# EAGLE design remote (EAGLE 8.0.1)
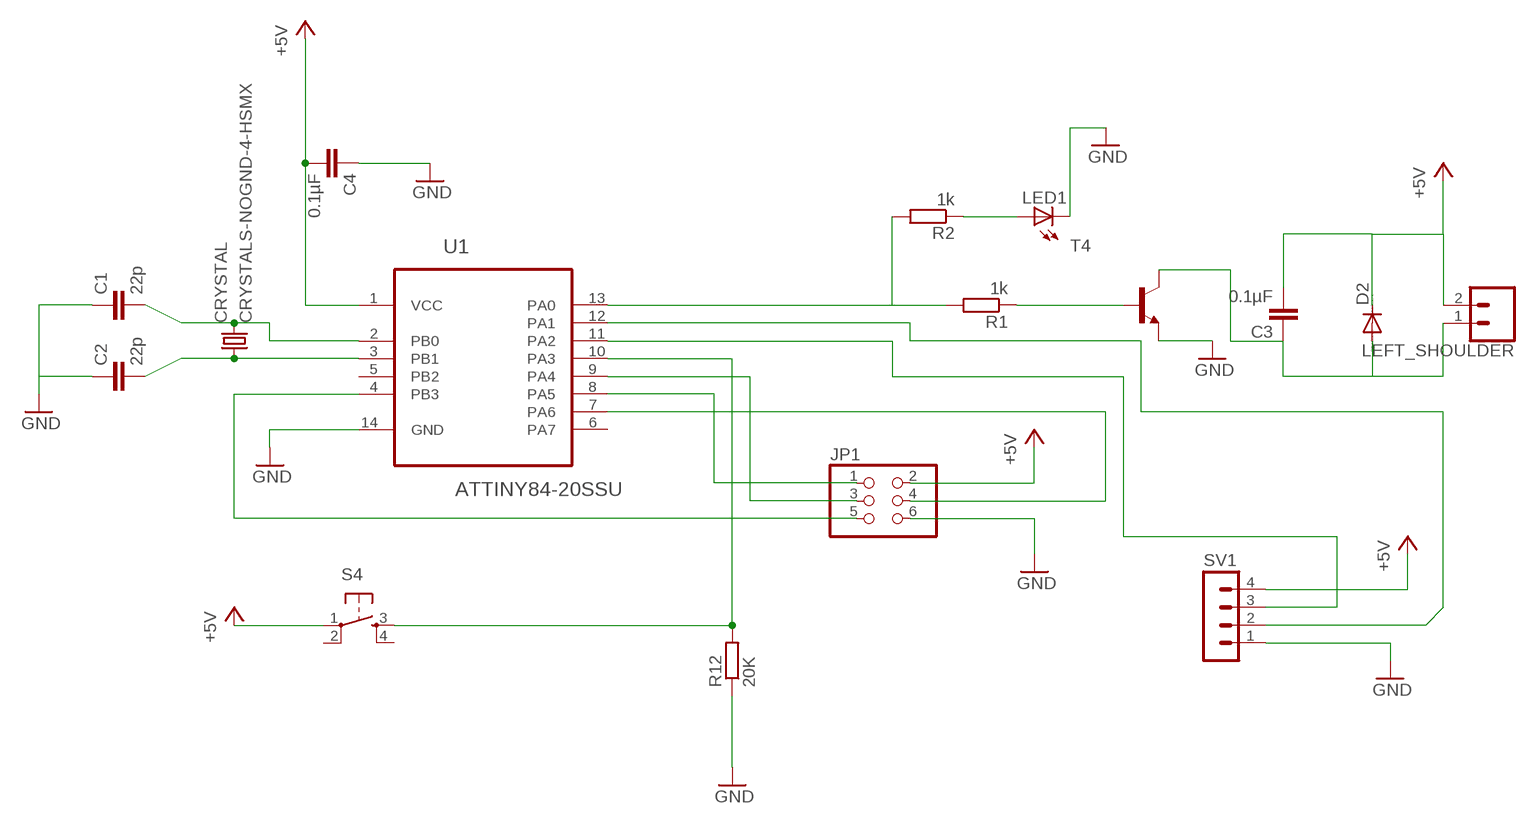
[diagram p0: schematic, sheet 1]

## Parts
C1  22p  C-EUC0603K  [C0603K]
C2  22p  C-EUC0603K  [C0603K]
C3  0.1µF  C-EUC0603K  [C0603K]
C4  0.1µF  C-EUC0603K  [C0603K]
CRYSTAL  CRYSTALS-NOGND-4-HSMX  [HC49-4-HSMX]
D2  DIODE-DO214AC  [DO214AC]
JP1  PINHD-2X3SMT  [2X03_SMT]
LED1  LEDCHIPLED_1206  [CHIPLED_1206]
LEFT_SHOULDER  CONN_02-JST-2MM-SMT  [JST-2-SMD]
R1  1k  R-EU_R1206  [R1206]
R2  1k  R-EU_R1206  [R1206]
R12  20K  R-EU_R1206  [R1206]
S4  LSG  [SCHURTER_LSG]
SV1  MA04-1  [MA04-1]
T4  -NPN-SOT23-EBC  [SOT23-EBC]
U1  ATTINY84-20SSU  [SOIC127P600X175-14N]

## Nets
+5V: C3.2 C4.2 D2.C JP1.2 LEFT_SHOULDER.2 S4.1(P) SV1.4 U1.1(VCC)
GND: C1.1 C2.1 C4.1 JP1.6 LED1.C R12.1 SV1.1 T4.E U1.14(GND)
N$1: JP1.3 U1.9(PA4)
N$2: C2.2 CRYSTAL.1 U1.3(PB1)
N$3: C3.1 D2.A LEFT_SHOULDER.1 T4.C
N$4: R1.1 T4.B
N$5: JP1.4 U1.7(PA6)
N$6: R12.2 S4.3(S) U1.10(PA3)
N$7: R1.2 R2.2 U1.13(PA0)
N$8: JP1.1 U1.8(PA5)
N$9: JP1.5 U1.4(PB3)
N$11: SV1.2 U1.12(PA1)
N$12: SV1.3 U1.11(PA2)
N$13: LED1.A R2.1
N$15: C1.2 CRYSTAL.2 U1.2(PB0)
Unconnected: S4.2(P1) S4.4(S1) U1.5(PB2) U1.6(PA7)

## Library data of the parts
C1-C4 = resistor:C-EU: CAPACITOR, European symbol
CRYSTAL = IQD-Frequency-Products:CRYSTALS-NOGND: CRYSTALS CAN NOT GROUNDED
D2 = diode:DIODE-: DIODE
JP1 = pinhead+:PINHD-2X3: PIN HEADER
LED1 = led:LED: LED
LEFT_SHOULDER = SparkFun-Connectors:CONN_02: Multi connection point. Often used as Generic Header-pin footprint for 0.1 inch spaced/style header connections; PROD_ID: CONN-11443
R1 R2 R12 = resistor:R-EU_: RESISTOR, European symbol
S4 = switch-omron:LSG
SV1 = con-lstb:MA04-1: PIN HEADER; OC_FARNELL: unknown; OC_NEWARK: unknown
T4 = transistor:*-NPN-: NPN Transistror BF959 corrected 2008.03.06
U1 = Atmel_By_element14_Batch_1-00:ATTINY84-20SSU: 8-bit Microcontroller with Bytes In-System Programmable Flash; MPN: ATTINY84-20SSU; OC_FARNELL: 1636955; OC_NEWARK: 03P2040; PACKAGE: SOIC-14; SUPPLIER: Atmel

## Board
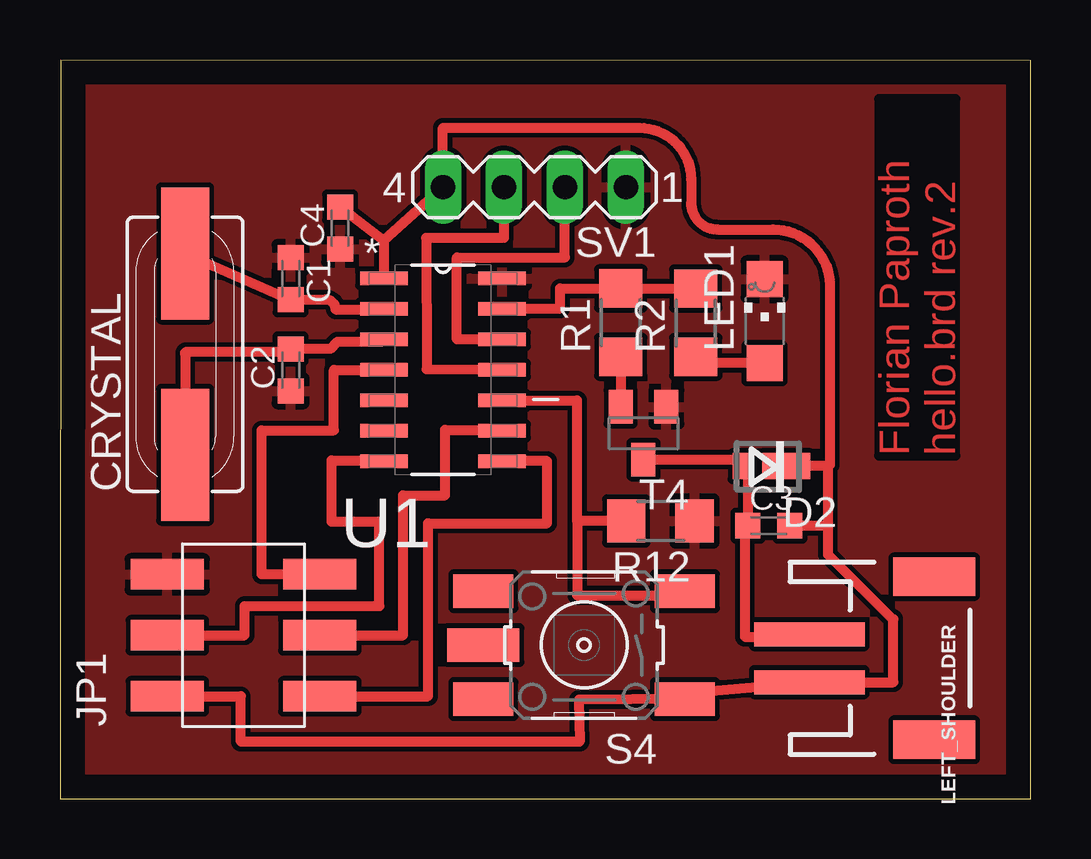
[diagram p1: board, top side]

Size 40.45 x 30.81 mm. Coordinates in mm from the lower left corner, seen from the top.
Outline: 0,0 40.45,0 40.44,30.78 0.04,30.81 0,0
Copper layers (1*16): Top 0.035mm / dielectric 1.5mm / Bottom 0.035mm
Design rules "default": minimum track width 10mil, minimum drill 24mil, track to track 8mil, track to pad 8mil, pad to pad 8mil, via to via 8mil, smd to smd 8mil, copper to edge 40mil, drill to drill 8mil, minimum pad ring 10mil, minimum via ring 8mil, stop-mask expansion 4mil, vias tented up to drill 0mil, thermal gap 10mil

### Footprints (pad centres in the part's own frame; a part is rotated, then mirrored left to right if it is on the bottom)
C0603K = smd 1.05 x 1.08: 1 -0.875,0; 2 0.875,0
HC49-4-HSMX = smd 5.5 x 2: 1 -4.2,0; 2 4.2,0
DO214AC = smd 0.813 x 1.092: A 1.321,0 | smd 2.007 x 1.092: C -0.508,0
2X03_SMT = smd 1.27 x 3.048: 1 -2.54,-3.175; 2 -2.54,3.175; 3 0,-3.175; 4 0,3.175; 5 2.54,-3.175; 6 2.54,3.175
CHIPLED_1206 = smd 1.5 x 1.5: A 0,-1.75; C 0,1.75
JST-2-SMD = smd 1 x 4.6: 1 -1,-3.7; 2 1,-3.7 | smd 1.6 x 3.4: NC1 -3.4,1.5; NC2 3.4,1.5
R1206 = smd 1.6 x 1.803: 1 -1.422,0; 2 1.422,0
SCHURTER_LSG = smd 2.5 x 1.4: 1 -4.2,2.25; 2 4.2,2.25; 3 -4.2,-2.25; 4 4.2,-2.25 | smd 3 x 1.4: 5 4.2,0
MA04-1 = drill 1.016 long: 1 -3.81,0; 2 -1.27,0; 3 1.27,0; 4 3.81,0
SOT23-EBC = smd 1 x 1.4: B 0.95,-1.1; C 0,1.1; E -0.95,-1.1
SOIC127P600X175-14N = smd 1.981 x 0.559: 1 -2.464,3.81; 2 -2.464,2.54; 3 -2.464,1.27; 4 -2.464,0; 5 -2.464,-1.27; 6 -2.464,-2.54; 7 -2.464,-3.81; 8 2.464,-3.81; 9 2.464,-2.54; 10 2.464,-1.27; 11 2.464,0; 12 2.464,1.27; 13 2.464,2.54; 14 2.464,3.81

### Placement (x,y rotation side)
C1  9.61,21.7 270 top
C2  9.61,17.89 90 top
C3  29.54,11.39 0 top
C4  11.67,23.81 90 top
CRYSTAL  5.21,18.54 90 top
D2  29.76,13.88 180 top
JP1  7.65,6.83 90 top
LED1  29.36,19.92 0 top
LEFT_SHOULDER  34.93,5.87 270 top
R1  23.37,19.86 90 top
R2  26.49,19.86 90 top
R12  25.02,11.6 180 top
S4  21.84,6.42 180 top
SV1  19.77,25.51 180 top
T4  24.31,15.25 180 top
U1  15.96,17.89 0 top

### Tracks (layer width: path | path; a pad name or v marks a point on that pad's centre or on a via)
+5V
  Top 0.406: 13.49,23.29 C4.2 | 13.49,23.29 U1.1 | 13.49,23.29 SV1.4 15.95,27.98 24.14,27.98 arc-90 26.3,25.82 26.3,24.85 arc90 27.39,23.75 29.72,23.75 arc-90 32.08,21.39 32.08,13.96 arc-90 32,13.88 | JP1.2 7.54,4.29 7.54,2.39 21.65,2.39 21.62,4.14 S4.1 26.4,4.44 LEFT_SHOULDER.2 34.72,4.87 34.72,7.5 34.68,7.5 32,10.19 32,11.39 | 32,11.39 C3.2 | 32,13.88 D2.C | 32,13.88 32,11.39
GND
  pour Top: -52.77,75.04 103.59,69.96 103.59,-43.07 -46.27,-43.07
N$1
  Top 0.406: JP1.3 14.29,6.83 14.29,12.66 16.05,12.66 16.05,15.39 18.42,15.39 U1.9
N$2
  Top 0.406: U1.3 13.41,19.07 11.56,19.07 11.25,18.77 C2.2 arc-90 9.48,18.64 5.28,18.64 arc90 5.21,18.56 CRYSTAL.1
N$3
  Top 0.406: T4.C 28.43,14.15 D2.A 28.66,13.88 C3.1 28.54,11.39 28.54,6.77 31.23,6.77 LEFT_SHOULDER.1
N$4
  Top 0.406: R1.1 T4.B
N$5
  Top 0.406: JP1.4 7.69,6.83 7.69,8.05 13.31,8.05 13.31,11.56 11.32,11.56 11.32,14.12 13.49,14.12 U1.7
N$6
  Top 0.406: U1.10 21.55,16.62 21.55,11.6 | 21.55,11.6 21.55,8.49 26.36,8.49 S4.3 | R12.2 21.55,11.6
N$7
  Top 0.406: U1.13 18.42,20.46 20.84,20.46 20.84,21.28 R1.2 R2.2
N$8
  Top 0.406: JP1.1 15.33,4.29 15.33,11.5 20.3,11.5 20.3,14.09 U1.8
N$9
  Top 0.406: JP1.5 8.41,9.37 8.41,15.37 11.41,15.37 11.41,17.89 U1.4
N$10
  Top 0.406: 9.6,20.52 9.6,20.74
N$11
  Top 0.406: U1.12 16.54,19.16 16.54,22.58 21.04,22.58 SV1.2
N$12
  Top 0.406: SV1.3 18.5,23.39 15.25,23.39 15.28,17.92 U1.11
N$13
  Top 0.406: LED1.A 26.5,18.17 26.5,17.93 26.49,17.93 R2.1
N$15
  Top 0.406: CRYSTAL.2 C1.2 arc90 C1.2 11.07,20.83 arc-90 11.48,20.41 13.48,20.41 arc90 U1.2

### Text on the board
Top: Florian Paproth / hello.brd rev.2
